FUNCTION_BLOCK p12_stanjeLucke
VAR_INPUT
	tipka: BOOL;
END_VAR
VAR_OUTPUT
	lucka: BOOL;
END_VAR
VAR
	detekcijaPozFronte: R_TRIG;
	tipkaPulz: BOOL;
	pomnilnaCelica: SR;
END_VAR

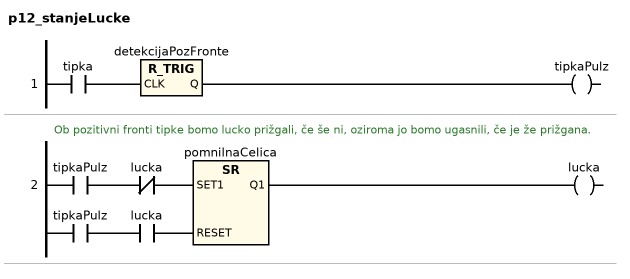
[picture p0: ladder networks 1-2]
// NETWORK 1
detekcijaPozFronte(CLK := tipka); // R_TRIG
tipkaPulz := detekcijaPozFronte.Q;

// NETWORK 2
// Ob pozitivni fronti tipke bomo lucko prižgali, če še ni, oziroma jo bomo ugasnili, če je že prižgana.
pomnilnaCelica(SET1 := tipkaPulz AND NOT lucka, RESET := tipkaPulz AND lucka); // SR
lucka := pomnilnaCelica.Q1;

END_FUNCTION_BLOCK
